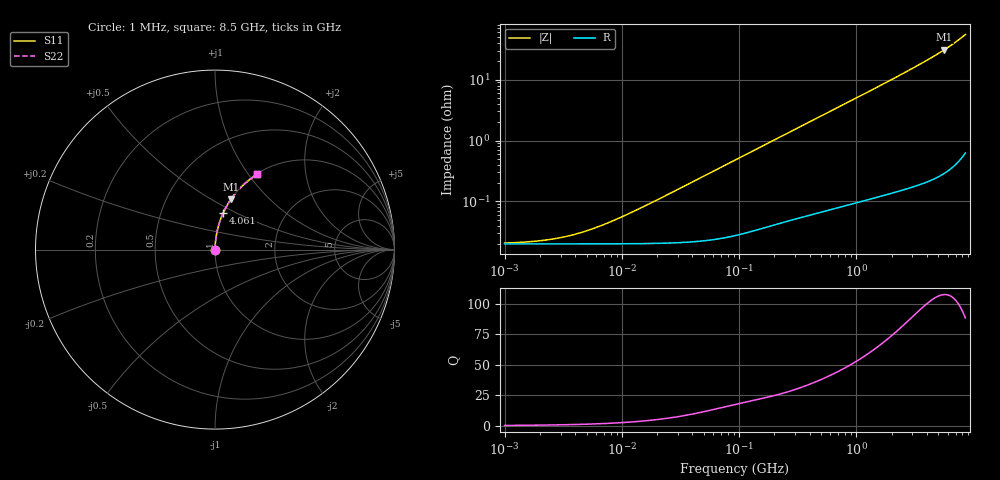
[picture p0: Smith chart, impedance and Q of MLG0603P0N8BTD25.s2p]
! S-Parameter Data Generated by TDK Corporation
! Copyright(C) 2025 TDK Corporation.
! All Rights Reserved.
! TDK P/N: MLG0603P0N8BTD25 (SMD / SMT Inductor (Coil))
! Property: L=0.8nH at 500MHz
! Size(LxWxT): 0.6x0.3x0.3mm
! Model Type: s2p (Touchstone File Format Version 1.0)
! Frequency: DC=Yes Start=1MHz Stop=8500MHz 198points Log-sweep
! Model Generated on Feb. 6, 2025
! Terms and conditions regarding TDK Simulation Models:
! 1)This simulation model is being provided solely for informational
!  purposes. Please refer to the specifications of the products in
!  terms of detailed characteristics of such products.
! 2)In no event shall TDK Corporation of any of its subsidiaries be
!  liable for any loss or damage arising, directly or indirectly,
!  from any information contained in this simulation model, including,
!  but not limited to loss or damages arising from any inaccuracies,
!  omissions or errors in connection with such information.
! 3)Any and all copyrights on this simulation model are owned by
!  TDK Corporation.  Duplication or redistribution of this simulation
!  model without prior written permission from TDK Corporation
!  is prohibited.
! 4)This simulation model is subject to any modification or change
!  without any prior notice.
! 5)Neither TDK Corporation nor any of its subsidiaries shall make any
!  warranty, express or implied, including but not limited to the
!  correctness, implied warranties of merchantability and fitness for
!  a particular purpose with respect to this simulation models.
! 6)The use of this simulation model shall be deemed to have consented
!  to the terms and conditions hereof.
! Port Assignments:
!  1 ---@@@--- 2
! Applicable Conditions:
!  Temperature = 25 degC
!  DC Bias Current = 0 A
!  Small Signal Operation
# Hz S MA R 50
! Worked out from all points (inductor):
!   197 points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, 1 MHz to 8.5 GHz, reference 50 ohm
!   read as one part in series: L = 827 pH near 12.09 MHz
!   highest Q = 107 at 5.61 GHz (marker M1), where L = 877 pH
!   S11 on the Smith chart (normalised r, x): 1 MHz: 1.00, +0.00; 4.061 GHz: 1.00, +0.42; 8.5 GHz: 1.01, +1.11
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1000000  0.0002066 14.6  0.9998 -0.0  0.9998 -0.0  0.0002066 14.6
1586648  0.0002163 22.4  0.9998 -0.0  0.9998 -0.0  0.0002163 22.4
2295435  0.0002329 30.8  0.9998 -0.0  0.9998 -0.0  0.0002329 30.8
3320851  0.0002642 40.8  0.9998 -0.0  0.9998 -0.0  0.0002642 40.8
4587603  0.0003113 50.0  0.9998 -0.0  0.9998 -0.0  0.0003113 50.0
6337562  0.0003855 58.7  0.9998 -0.0  0.9998 -0.0  0.0003855 58.7
8755050  0.0004973 66.2  0.9998 -0.0  0.9998 -0.0  0.0004973 66.2
1.26661e7  0.0006883 72.9  0.9998 -0.0  0.9998 -0.0  0.0006883 72.9
2.10461e7  0.001112 79.3  0.9998 -0.1  0.9998 -0.1  0.001112 79.3
9.219544e7  0.004765 86.4  0.9997 -0.3  0.9997 -0.3  0.004765 86.4
4.229561e8  0.0213 87.1  0.9992 -1.2  0.9992 -1.2  0.0213 87.1
1.016736e9  0.05074 86.0  0.9978 -2.9  0.9978 -2.9  0.05074 86.0
1.404574e9  0.07002 85.1  0.9964 -4.0  0.9964 -4.0  0.07002 85.1
1.940355e9  0.09684 83.7  0.994 -5.6  0.994 -5.6  0.09684 83.7
2.939772e9  0.1478 80.9  0.9873 -8.5  0.9873 -8.5  0.1478 80.9
4.061159e9  0.2072 77.5  0.9762 -12.0  0.9762 -12.0  0.2072 77.5
4.884749e9  0.2528 74.8  0.9651 -14.6  0.9651 -14.6  0.2528 74.8
5.610304e9  0.2947 72.3  0.9528 -17.1  0.9528 -17.1  0.2947 72.3
6.44363e9  0.3451 69.3  0.9353 -20.2  0.9353 -20.2  0.3451 69.3
7.066863e9  0.3846 66.8  0.9193 -22.6  0.9193 -22.6  0.3846 66.8
7.750377e9  0.4297 64.0  0.8985 -25.4  0.8985 -25.4  0.4297 64.0
8.5e9  0.4814 60.6  0.8711 -28.8  0.8711 -28.8  0.4814 60.6
